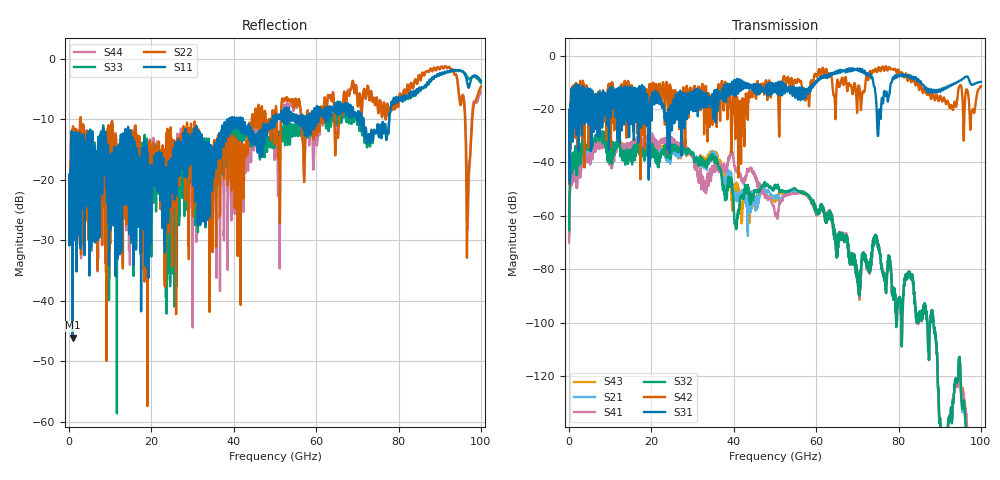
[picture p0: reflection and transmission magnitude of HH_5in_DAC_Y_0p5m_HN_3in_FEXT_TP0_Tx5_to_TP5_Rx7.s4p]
# GHz S RI R 45
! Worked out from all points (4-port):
!   4000 points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, 25 MHz to 100 GHz, reference 45 ohm
!   strongest paths, dB at 25 MHz, 25.02 GHz, 50.02 GHz, 75.03 GHz, 100 GHz:
!     S31: -35.1, -26.8, -12.5, -30.1, -9.8
!     S42: -34.9, -18.5, -12.5, -4.7, -11.5
!     S32: -65.4, -34.5, -48.6, -71.4, -178.4
!     S41: -70.0, -31.7, -59.0, -71.3, -178.8
!     S21: -67.6, -35.5, -52.5, -71.3, -176.5
!     S43: -67.4, -34.1, -54.0, -71.3, -179.9
!   lowest |S11| = -46.1 dB at 900 MHz (marker M1), VSWR 1.01, Z = 44.6 + j0.181 ohm
!   |S11| at or under -10 dB: start of sweep to 38.97 GHz; 42.22 GHz to 49.54 GHz (7.317 GHz wide, 16 % of centre); 71.52 GHz to 77.73 GHz (6.209 GHz wide, 8.32 % of centre)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
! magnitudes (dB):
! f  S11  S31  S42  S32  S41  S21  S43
! 25 MHz  -24.0  -35.1  -34.9  -65.4  -70.0  -67.6  -67.4
! 900 MHz  -46.1  -32.2  -20.6  -37.9  -41.7  -39.9  -39.9
! 39.4 GHz  -10.9  -13.1  -29.0  -45.9  -35.2  -44.4  -49.1
! 70.1 GHz  -9.8  -5.0  -15.0  -81.8  -81.4  -81.5  -81.7
! 75.22 GHz  -12.9  -23.9  -4.3  -71.9  -71.7  -71.8  -71.8
! 96.9 GHz  -4.6  -8.2  -14.2  -172.2  -161.8  -161.8  -167.8
! 100 GHz  -3.6  -9.8  -11.5  -178.4  -178.8  -176.5  -179.9
